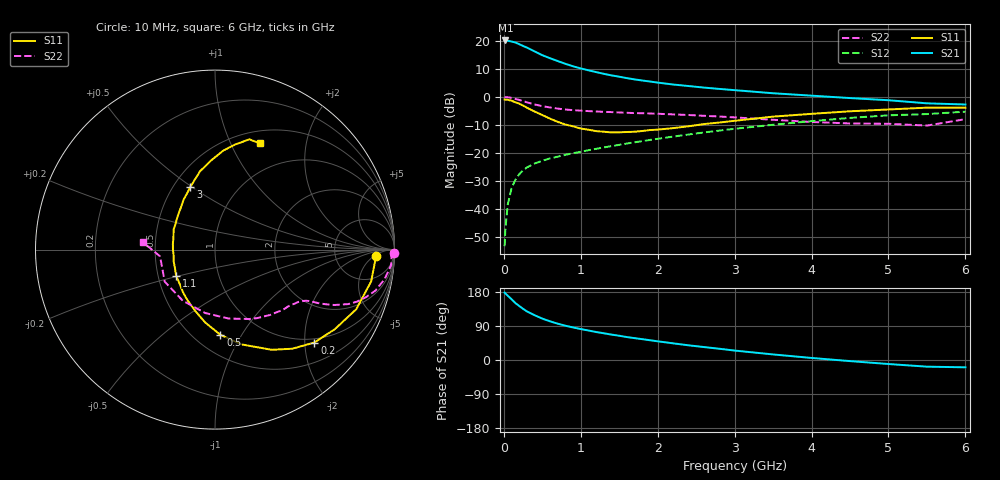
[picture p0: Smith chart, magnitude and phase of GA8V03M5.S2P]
! Infineon Technologies  Discrete & RF Semiconductors
! BF775
! Si NPN RF Bipolar Junction Transistor in SOT23
! VCE = 8 V  IC = 3.5 mA
! Common Emitter S-Parameters:  May  1996
# GHz  S  MA  R  50
!  f  S11  S21  S12  S22
! GHz  MAG  ANG  MAG  ANG  MAG  ANG  MAG  ANG
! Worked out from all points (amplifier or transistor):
!   36 points, 10 MHz to 6 GHz, reference 50 ohm
!   highest |S21| = 20.1 dB at 20 MHz (marker M1)
!   |S21| within 3 dB of that: start of sweep to 333.7 MHz
!   unconditionally stable (mu >= 1): 981.1 MHz to 3.137 GHz
!   at 250 MHz: K = 0.38, MSG = 22.1 dB, |S12| = -26.2 dB
!   at 1.4 GHz: K = 1.10, MAG = 10.6 dB, |S12| = -17.5 dB
!   at 6 GHz: K = 0.92, MSG = 1.3 dB, |S12| = -5.3 dB
!   S11 on the Smith chart (normalised r, x): 10 MHz: 16, -6; 200 MHz: 0.91, -2.21; 500 MHz: 0.66, -0.81; 1.1 GHz: 0.62, -0.19; 3 GHz: 0.61, +0.49; 6 GHz: 0.64, +1.29
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0.01  0.8992 -2.3  10.01 177.9  0.0022 90.3  0.9962 -1.0
0.02  0.8936 -4.5  10.11 175.6  0.0044 91.5  0.9837 -2.0
0.05  0.888 -11.5  10.03 169.8  0.012 83.9  0.985 -5.1
0.1  0.8541 -22.9  9.671 160.4  0.0236 77.2  0.9591 -9.9
0.15  0.8014 -33.6  9.305 150.3  0.0334 71.5  0.9229 -14.3
0.2  0.7579 -43.1  8.669 142.6  0.042 67.8  0.882 -17.5
0.25  0.6999 -52.1  8.071 135.0  0.0492 63.3  0.8413 -20.2
0.3  0.6414 -60.5  7.542 128.2  0.0554 61.2  0.8006 -22.3
0.4  0.5484 -74.4  6.45 118.2  0.0652 57.2  0.7331 -24.9
0.5  0.4756 -86.4  5.518 109.2  0.0731 54.9  0.6838 -26.4
0.6  0.4101 -97.6  4.879 102.1  0.0803 54.0  0.6474 -27.4
0.7  0.3593 -107.8  4.346 95.9  0.0863 53.9  0.6188 -28.1
0.8  0.3224 -118.1  3.88 90.5  0.0928 53.9  0.5965 -28.7
1.1  0.2606 -146.3  2.972 77.8  0.1124 54.8  0.5587 -31.2
1.3  0.2399 -163.4  2.574 70.5  0.1261 55.3  0.5418 -33.1
1.6  0.2371 172.2  2.157 60.5  0.1478 55.8  0.5212 -36.6
2.2  0.278 138.8  1.661 44.0  0.1964 54.8  0.488 -46.0
3  0.3755 111.5  1.318 24.9  0.2704 49.9  0.4314 -63.7
3.5  0.4451 100.7  1.161 14.7  0.3188 45.1  0.3913 -78.9
4.5  0.5544 85.1  0.953 -2.9  0.4224 33.4  0.3364 -122.4
5.5  0.6433 72.7  0.768 -17.6  0.4947 17.8  0.3085 -173.0
6  0.6424 67.2  0.732 -19.3  0.5463 13.5  0.4018 174.3
